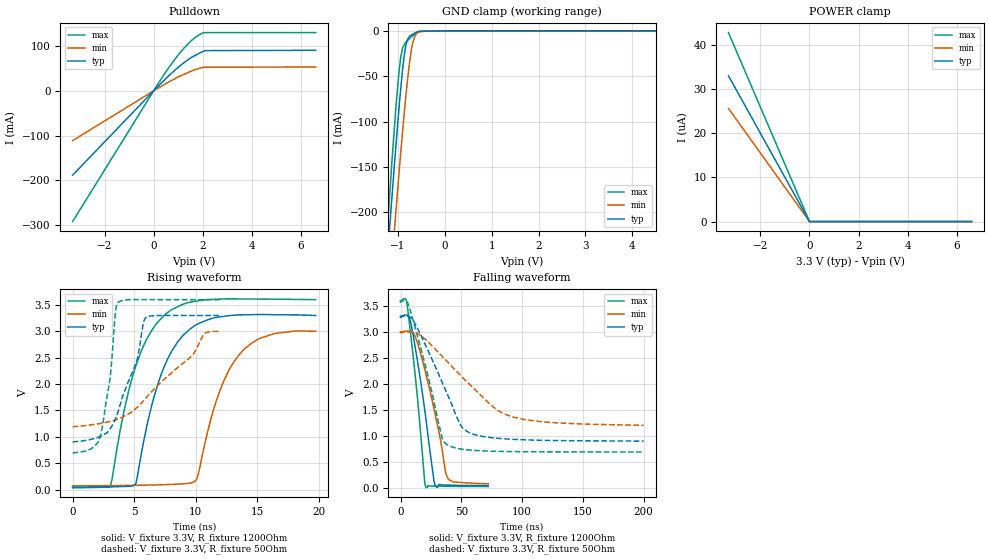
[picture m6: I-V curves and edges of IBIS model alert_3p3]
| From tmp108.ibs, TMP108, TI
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|   alert_3p3 Model
[Model]   alert_3p3
Model_type   Open_drain
Polarity   Non-Inverting
Vmeas = 1.65
Vref = 3.3
Cref = 2pF
Rref = 1200
|   typ   min   max
C_comp   7.138e-13   7.020e-13   7.777e-13
| Where nom  PVT is Nominal Process, 3.3V, 27C
|   Fast PVT is Strong Process,  3.6V, -40C
|   Slow PVT is Weak Process,   3V, 125C
[Voltage Range]   3.3   3   3.6
|Ambient Temperature   25   125   -40
|Junction Temperature
[Temperature Range]   27   125   -40
[Pullup Reference]   3.3   3   3.6
[Pulldown Reference]   0   0   0
[Power Clamp Reference]   3.3   3   3.6
[GND Clamp Reference]   0   0   0
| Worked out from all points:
|   slope of the pulldown table from 0 to 0.495 V, typ, clamps not added: 18.2 ohm
|   GND clamp passes 1 mA (typ) near -0.58 V on its own axis
|   falling waveform, V_fixture 3.3V, R_fixture 1200Ohm: 20-80 % time 11.8ns typ, 16.2ns min, 8.96ns max; typ from 3.3 V to 0.051 V
|   rising waveform, V_fixture 3.3V, R_fixture 1200Ohm: 20-80 % time 2.52ns typ, 2.54ns min, 2.52ns max; typ from 0.048 V to 3.3 V
|   falling waveform, V_fixture 3.3V, R_fixture 50Ohm: 20-80 % time 26.8ns typ, 46.2ns min, 18.3ns max; typ from 3.3 V to 0.906 V
|   rising waveform, V_fixture 3.3V, R_fixture 50Ohm: 20-80 % time 1.96ns typ, 4.78ns min, 878ps max; typ from 0.904 V to 3.3 V
[Pulldown]
|   Voltage   I(typ)   I(min)   I(max)
-3.3V     -188.7mA   -111.5mA   -292.4mA
453.6mV   25.01mA    14.64mA    38.91mA
1.044V    54.46mA    32.28mA    83.14mA
1.526V    74.28mA    43.87mA    111.7mA
1.706V    79.6mA     47.49mA    120mA
1.948V    86.38mA    51.46mA    128.3mA
2.128V    89.89mA    52.7mA     130.2mA
6.6V      90.63mA    53.27mA    130.2mA
[GND Clamp]
|   Voltage   I(typ)   I(min)   I(max)
-3.3V     -1.734A    -1.745A    -1.76A
-1.247V   -268.7mA   -335.1mA   -237.1mA
-1.119V   -179.8mA   -249.4mA   -140.5mA
-1.105V   -170.3mA   -240.7mA   -130.4mA
-1.037V   -125mA     -197.3mA   -82.97mA
-979.2mV  -88.95mA   -160.8mA   -48.22mA
-939.6mV  -65.7mA    -136.4mA   -30.1mA
-858mV    -25.64mA   -88.69mA   -15.16mA
-792mV    -9.536mA   -54.16mA   -10.66mA
-711mV    -4.641mA   -21.33mA   -6.755mA
-590.7mV  -1.13mA    -2.638mA   -2.203mA
6.6V      0A         0A         0A
[POWER Clamp]
|   Voltage   I(typ)   I(min)   I(max)
-3.3V     32.99uA    25.62uA    42.76uA
-3mV      30.11nA    25.43nA    38.95nA
-33.83fV  0A         0A         0A
6.6V      0A         0A         0A
[Ramp]
R_load = 1200
|   typ   min   max
dV/dt_r   1.95114/2.52017e-09   1.75607/2.53566e-09   2.13966/2.52391e-09
dV/dt_f   1.95111/1.18064e-08   1.75567/1.62762e-08   2.13966/8.96403e-09
[Falling Waveform]
V_fixture = 3.3V
V_fixture_min = 3V
V_fixture_max = 3.6V
R_fixture = 1200Ohm
|   Time   V(typ)   V(min)   V(max)
0s        3.3V       3V         3.6V
4.17ns    3.327V     3.016V     3.636V
5.7ns     3.325V     3.017V     3.477V
7.69ns    3.251V     3.014V     3.09V
12.02ns   2.716V     2.914V     2.18V
20.59ns   1.385V     2.223V     36.03mV
28.57ns   54.49mV    1.415V     40.84mV
36.81ns   63.49mV    336.7mV    37.08mV
39.15ns   60.83mV    181.7mV    36.58mV
72.09ns   50.85mV    88.01mV    34.45mV
[Rising Waveform]
V_fixture = 3.3V
V_fixture_min = 3V
V_fixture_max = 3.6V
R_fixture = 1200Ohm
|   Time   V(typ)   V(min)   V(max)
0s        48.09mV    73.21mV    33.9mV
3ns       51.98mV    75.83mV    46.27mV
4.21ns    60.43mV    78.67mV    1.526V
5.12ns    103.1mV    81.51mV    2.335V
6.45ns    1.617V     87.58mV    3.026V
7.67ns    2.451V     96.09mV    3.347V
10.09ns   3.131V     202.5mV    3.573V
11.99ns   3.274V     1.894V     3.61V
13.96ns   3.313V     2.666V     3.613V
19.75ns   3.3V       3V         3.6V
[Falling Waveform]
V_fixture = 3.3V
V_fixture_min = 3V
V_fixture_max = 3.6V
R_fixture = 50Ohm
|   Time   V(typ)   V(min)   V(max)
0s        3.3V       3V         3.6V
7.18ns    3.296V     3.001V     3.479V
21.69ns   2.691V     2.831V     2.238V
34.4ns    2.026V     2.53V      949.8mV
38.46ns   1.81V      2.431V     833.3mV
50.15ns   1.188V     2.148V     752.1mV
61.65ns   1.024V     1.886V     725.4mV
80.09ns   958.7mV    1.495V     708.7mV
101.4ns   930.6mV    1.322V     701.6mV
200ns     905.6mV    1.208V     696.3mV
[Rising Waveform]
V_fixture = 3.3V
V_fixture_min = 3V
V_fixture_max = 3.6V
R_fixture = 50Ohm
|   Time   V(typ)   V(min)   V(max)
0s        903.7mV    1.192V     696.1mV
2.17ns    1.001V     1.25V      936.8mV
3.04ns    1.151V     1.291V     2.101V
3.5ns     1.352V     1.322V     3.398V
3.73ns    1.503V     1.343V     3.556V
5.28ns    2.499V     1.567V     3.601V
5.96ns    3.266V     1.737V     3.6V
9.77ns    3.3V       2.556V     3.6V
10.83ns   3.3V       2.974V     3.6V
12ns      3.3V       3V         3.6V
